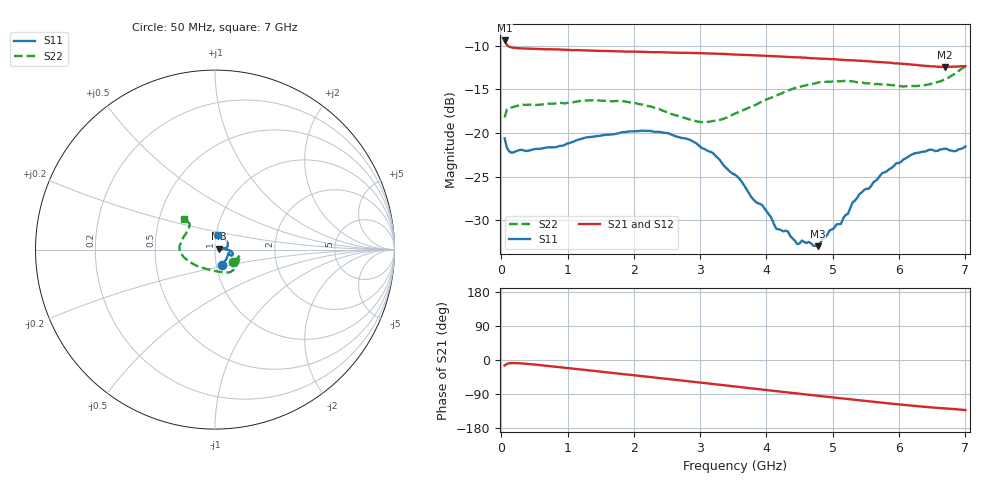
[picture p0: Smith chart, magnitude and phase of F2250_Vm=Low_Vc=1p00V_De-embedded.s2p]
! Integrated Device Technology
! Corporate Headquarters
! 6024 Silver Creek Valley Road
! San Jose, CA 95138  USA
! Phone:  1-408-284-8200
! Toll Free:  1-800-223-1366
! Webpage:  http://www.idt.com/
! Timing and RF Division
! 515 Groton Road, Suite 102
! Westford, MA 01886-6024
! Device:  F2250
! Description: Voltage Variable RF Attenuator
! Frequency:  50.0 -  6000.00 MHz
! Package:  3x3 mm Thin QFN Plastic Package: 16 pin
! Ports:  2 RF, 3 DC
!  Pin  1  = GND
!  Pin  2  = NC
!  Pin  3  = RF1  = Port 1
!  Pin  4  = NC
!  Pin  5  = GND
!  Pin  6  = GND
!  Pin  7  = GND
!  Pin  8  = GND
!  Pin  9  = NC
!  Pin 10  = RF2  = Port 2
!  Pin 11  = NC
!  Pin 12  = GND
!  Pin 13  = GND
!  Pin 14  = VCNTRL
!  Pin 15  = VDD
!  Pin 16  = VMODE
! Vcntrl:  1.000 Volts
! Vmode:  +0.000 Volts
! Vdd:  +3.30  Volts
! Current:  1.188 mA
! Data:  The device was measured on a the F2250 evaluation board which has
!  individual transmission lines to the RF pins.  Data was collected
!  using a calibrated network analyzer.  The evaluation board was
!  de-embedded using a TRL calibration technique.
!  The reference plane is the edge of the package pin.
! Misc:  SN 10
!  Action Tracker AT0258
! Date Measured:  2014-11-26
! Date:  2015-10-15  MJV
! Note:
!  Integrated Device Technology supplies this data as a sample of measured
!  data at the package pin for this product.  Your particular data for this
!  product may vary.
!  Data was taken at 25 degrees C.
!  Integrated Device Technology reserves the right to change this data at anytime.
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# GHz S dB R 50
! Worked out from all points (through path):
!   201 points, 50 MHz to 7 GHz, reference 50 ohm
!   highest |S21| = -9.39 dB at 50 MHz (marker M1); lowest = -12.4 dB at 6.687 GHz (marker M2)
!   group delay of S21, straight-line fit = 52.5 ps
!   lowest |S11| = -32.9 dB at 4.776 GHz (marker M3), VSWR 1.05, Z = 52.2 + j0.503 ohm
!   |S11| at or under -10 dB: start of sweep to end of sweep
!   |S22| runs from -18.8 to -12.3 dB; largest |S21 - S12| = 0.00084
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0.05  -20.59 -64.1  -9.39 -14.2  -9.39 -14.2  -18.22 -33.5
0.08475  -21.69 -38.2  -9.92 -10.1  -9.95 -10.2  -17.28 -18.4
0.15425  -22.25 -23.3  -10.19 -8.1  -10.20 -8.1  -17.07 -13.2
1.2315  -20.61 -19.8  -10.53 -25.6  -10.52 -25.6  -16.28 -41.4
2.37825  -19.85 -12.4  -10.74 -47.3  -10.73 -47.4  -17.24 -68.7
3.0385  -21.75 -3.6  -10.87 -60.3  -10.86 -60.3  -18.75 -100.8
3.525  -24.76 2.7  -11.01 -69.9  -11.01 -69.9  -17.77 -131.0
3.803  -27.61 7.5  -11.09 -75.4  -11.09 -75.4  -16.86 -144.6
3.942  -28.32 9.2  -11.13 -78.1  -11.14 -78.1  -16.35 -151.1
4.1505  -30.99 13.5  -11.20 -82.2  -11.19 -82.2  -15.69 -159.2
4.32425  -31.28 14.4  -11.27 -85.6  -11.28 -85.5  -15.13 -164.4
4.46325  -32.70 15.2  -11.32 -88.3  -11.32 -88.3  -14.80 -168.2
4.53275  -32.30 14.2  -11.34 -89.7  -11.35 -89.7  -14.64 -170.3
4.7065  -32.91 15.7  -11.43 -93.0  -11.43 -93.0  -14.35 -174.0
4.776  -32.95 12.3  -11.47 -94.3  -11.47 -94.3  -14.21 -175.4
4.94975  -31.16 7.1  -11.52 -97.7  -11.52 -97.7  -14.11 -179.2
5.1235  -30.39 5.6  -11.60 -101.0  -11.60 -101.0  -14.06 176.8
5.4015  -26.99 4.2  -11.71 -106.3  -11.71 -106.3  -14.18 170.3
5.85325  -24.12 8.4  -11.93 -114.6  -11.94 -114.7  -14.49 158.8
6.2355  -22.32 19.8  -12.18 -121.3  -12.17 -121.4  -14.61 146.1
6.68725  -21.79 45.6  -12.43 -127.7  -12.42 -127.7  -13.81 134.5
7  -21.52 77.6  -12.33 -132.1  -12.32 -132.2  -12.30 134.5
